[IBIS VER]   4.1
[File Name]   f29h85xrfs.ibs
[File Rev]   1.0
[Date]   May 06, 2024
[Source]   File originated at Texas Instruments
[Copyright]   (c) 2012, Texas Instruments Inc.
[Component]   f29h85xrfs
[Manufacturer]  Texas Instruments
[Package]
| Variable   Typ   Min   Max
R_pkg   2.68E-01   1.13E-01   3.72E-01
L_pkg   6.91E-09   5.05E-09   8.22E-09
C_pkg   1.08E-13   7.65E-14   2.06E-13
[Pin]   signal_name   model_name   R_pin   L_pin   C_pin
1   GPIO15   BQ33100HYPBFZ_PMB_5FS_LC_7LM   2.88E-01   7.82E-09   2.03E-13
2   GPIO16   BCF33100DSHYPBFZ_USF_7LM   2.89E-01   7.74E-09   1.00E-13
3   VDDIO   NC   2.81E-01   7.58E-09   9.82E-14
4   GPIO17   BCF33100DSHYPBFZ_USF_7LM   2.78E-01   7.47E-09   9.65E-14
5   GPIO19   BCF33100DSHYPBFZ_USF_7LM   2.72E-01   7.32E-09   9.48E-14
6   VDD   NC   1.62E-01   6.27E-09   9.54E-14
7   GPIO34   BCF33100DSHYPBFZ_USF_7LM   3.01E-01   7.40E-09   9.18E-14
8   VDD   NC   1.84E-01   6.29E-09   9.29E-14
9   VDDIO   NC   3.72E-01   7.84E-09   8.90E-14
10   GPIO18   BQ33100HYPBFZ_PMB_5FS_LC_7LM   3.58E-01   7.63E-09   8.73E-14
11   GPIO22   BQ33100HYPBFZ_PMB_5FS_LC_7LM   3.52E-01   7.49E-09   8.55E-14
12   B11,GPIO235   BCF33100DSHYPBFZ_USF_7LM   3.46E-01   7.35E-09   8.38E-14
13   B10,GPIO234   BCF33100DSHYPBFZ_USF_7LM   3.33E-01   7.15E-09   8.20E-14
14   B9,GPIO233   BCF33100DSHYPBFZ_USF_7LM   3.33E-01   7.06E-09   8.04E-14
15   B8,GPIO232   BCF33100DSHYPBFZ_USF_7LM   3.22E-01   6.87E-09   7.86E-14
16   A8,GPIO226   BCF33100DSHYPBFZ_USF_7LM   3.17E-01   6.74E-09   7.69E-14
17   A7/E25,GPIO225   BCF33100DSHYPBFZ_USF_7LM   3.23E-01   6.70E-09   2.02E-13
18   A6/E24,GPIO224   BCF33100DSHYPBFZ_USF_7LM   3.12E-01   6.52E-09   1.97E-13
19   VDDA   NC   1.91E-01   5.46E-09   2.00E-13
20   VSSA   NC   1.86E-01   5.50E-09   2.05E-13
21   B5/D31   ICF33SHYPB_LC_7LM   3.28E-01   6.83E-09   7.70E-14
22   B4/D30   ICF33SHYPB_LC_7LM   3.14E-01   6.81E-09   7.85E-14
23   A5/D29   ICF33SHYPB_LC_7LM   3.02E-01   6.78E-09   8.01E-14
24   A4/D28   ICF33SHYPB_LC_7LM   2.90E-01   6.77E-09   8.17E-14
25   B3/D27   ICF33SHYPB_LC_7LM   2.80E-01   6.77E-09   8.32E-14
26   B2/D26   ICF33SHYPB_LC_7LM   2.71E-01   6.79E-09   8.48E-14
27   A3/D25   ICF33SHYPB_LC_7LM   2.64E-01   6.82E-09   8.64E-14
28   A2/D24   ICF33SHYPB_LC_7LM   2.60E-01   6.87E-09   8.81E-14
29   VREFLOAB   NC   1.49E-01   5.99E-09   9.17E-14
30   VREFHIAB   NC   1.13E-01   5.76E-09   9.54E-14
31   A15/B15/C15/D15/E15   ICF33SHYPB_LC_7LM   2.57E-01   7.11E-09   9.30E-14
32   A14/B14/C14/D14/E14   ICF33SHYPB_LC_7LM   2.60E-01   7.22E-09   9.47E-14
33   B1/C27   ICF33SHYPB_LC_7LM   2.65E-01   7.35E-09   9.64E-14
34   B0/C26/VDAC   ICF33SHYPB_LC_7LM   2.72E-01   7.50E-09   9.82E-14
35   A1/C25   ICF33SHYPB_LC_7LM   2.80E-01   7.67E-09   9.99E-14
36   A0/C24/DACA_OUT   ICF33SHYPB_LC_7LM   2.91E-01   7.85E-09   2.03E-13
37   C0/E28   ICF33SHYPB_LC_7LM   2.91E-01   7.89E-09   2.05E-13
38   C1/E29   ICF33SHYPB_LC_7LM   2.80E-01   7.70E-09   1.01E-13
39   D0/B24   ICF33SHYPB_LC_7LM   2.70E-01   7.53E-09   9.89E-14
40   D1/B25   ICF33SHYPB_LC_7LM   2.63E-01   7.38E-09   9.72E-14
41   E0/A24/DACC_OUT   ICF33SHYPB_LC_7LM   2.58E-01   7.24E-09   9.54E-14
42   E1/A25   ICF33SHYPB_LC_7LM   2.55E-01   7.13E-09   9.37E-14
43   C2/E30   ICF33SHYPB_LC_7LM   2.54E-01   7.03E-09   9.20E-14
44   C3/E31   ICF33SHYPB_LC_7LM   2.56E-01   6.96E-09   9.04E-14
45   VREFLOCDE   NC   1.50E-01   5.94E-09   9.08E-14
46   VREFHICDE   NC   1.13E-01   5.52E-09   9.12E-14
47   C4   ICF33SHYPB_LC_7LM   2.67E-01   6.79E-09   8.54E-14
48   C5   ICF33SHYPB_LC_7LM   2.76E-01   6.77E-09   8.38E-14
49   D2/B26   ICF33SHYPB_LC_7LM   2.86E-01   6.77E-09   8.23E-14
50   D3/B27   ICF33SHYPB_LC_7LM   2.97E-01   6.78E-09   8.07E-14
51   E2/A26   ICF33SHYPB_LC_7LM   3.10E-01   6.80E-09   7.91E-14
52   E3/A27   ICF33SHYPB_LC_7LM   3.24E-01   6.83E-09   7.75E-14
53   VSSA   NC   1.84E-01   5.52E-09   2.06E-13
54   VDDA   NC   1.89E-01   5.47E-09   2.02E-13
55   D5/B29,GPIO241   BCF33100DSHYPBFZ_USF_7LM   2.67E-01   6.15E-09   1.98E-13
56   E4/A28,GPIO246   BCF33100DSHYPBFZ_USF_7LM   2.67E-01   6.24E-09   2.03E-13
57   E5/A29,GPIO247   BCF33100DSHYPBFZ_USF_7LM   2.68E-01   6.35E-09   7.71E-14
58   C8,GPIO238   BCF33100DSHYPBFZ_USF_7LM   2.72E-01   6.47E-09   7.88E-14
59   C9,GPIO239   BCF33100DSHYPBFZ_USF_7LM   2.77E-01   6.60E-09   8.05E-14
60   D6/B30,GPIO242   BCF33100DSHYPBFZ_USF_7LM   2.83E-01   6.75E-09   8.22E-14
61   D7/B31,GPIO243   BCF33100DSHYPBFZ_USF_7LM   2.91E-01   6.91E-09   8.40E-14
62   E6/A30,GPIO248   BCF33100DSHYPBFZ_USF_7LM   3.01E-01   7.08E-09   8.57E-14
63   E7/A31,GPIO249   BCF33100DSHYPBFZ_USF_7LM   3.11E-01   7.26E-09   8.75E-14
64   GPIO222/TDI   BCF33100DSHYPBFZ_USF_7LM   3.11E-01   7.35E-09   8.92E-14
65   GPIO223/TDO   BCPF335585DSHYPBFZ_USF_7LM   3.23E-01   7.55E-09   9.10E-14
66   VDDIO   NC   3.35E-01   7.74E-09   9.28E-14
67   VDD   NC   1.42E-01   6.14E-09   1.00E-13
68   VDD3VFL   NC   1.39E-01   6.20E-09   1.01E-13
69   TMS   BCF3355DSHYPBFZ_TMS_USF_7LM   3.36E-01   8.02E-09   9.78E-14
70   TCK   IQ0442FS_40P60P_3X2_USF_7LM   3.49E-01   8.22E-09   9.96E-14
71   VDD   NC   1.47E-01   6.54E-09   1.07E-13
72   VDDIO   NC   2.87E-01   7.86E-09   2.05E-13
73   GPIO41   BCF33100DSHYPBFZ_CORNER_USF_7LM   2.88E-01   7.82E-09   2.03E-13
74   GPIO219/ERRORSTS   BCF33100DSHYPBFZ_CORNER_USF_7LM   3.00E-01   7.84E-09   1.00E-13
75   GPIO49   BCF33100DSHYPBFZ_USF_7LM   2.91E-01   7.67E-09   9.83E-14
76   GPIO50   BCF33100DSHYPBFZ_USF_7LM   2.83E-01   7.52E-09   9.66E-14
77   GPIO51   BCF33100DSHYPBFZ_USF_7LM   2.76E-01   7.37E-09   9.49E-14
78   GPIO52   BCF33100DSHYPBFZ_USF_7LM   2.74E-01   7.26E-09   9.32E-14
79   GPIO53   BCF33100DSHYPBFZ_USF_7LM   2.69E-01   7.12E-09   9.15E-14
80   GPIO54   BCF33100DSHYPBFZ_USF_7LM   2.66E-01   7.01E-09   8.98E-14
81   VDDIO   NC   2.64E-01   6.90E-09   8.81E-14
82   GPIO56   BCF33100DSHYPBFZ_USF_7LM   2.65E-01   6.82E-09   8.64E-14
83   VDD3VFL   NC   1.14E-01   5.41E-09   8.90E-14
84   GPIO57   BCF33100DSHYPBFZ_USF_7LM   2.65E-01   6.65E-09   8.31E-14
85   GPIO58   BCF33100DSHYPBFZ_USF_7LM   2.66E-01   6.56E-09   8.15E-14
86   GPIO59   BCF3385DSHYPBFZ_USF_7LM   2.68E-01   6.49E-09   7.98E-14
87   VDD   NC   1.14E-01   5.05E-09   8.26E-14
88   GPIO60   BCF33100DSHYPBFZ_USF_7LM   2.72E-01   6.35E-09   7.65E-14
89   GPIO61   BCF33100DSHYPBFZ_USF_7LM   2.69E-01   6.23E-09   2.01E-13
90   GPIO62   BCF33100DSHYPBFZ_USF_7LM   2.71E-01   6.16E-09   1.97E-13
91   GPIO63   BCF33100DSHYPBFZ_USF_7LM   2.73E-01   6.18E-09   1.97E-13
92   GPIO64   BCF3385DSHYPBFZ_USF_7LM   2.77E-01   6.30E-09   2.01E-13
93   GPIO65   BCF33100DSHYPBFZ_USF_7LM   2.82E-01   6.43E-09   7.66E-14
94   GPIO66   BCF33100DSHYPBFZ_USF_7LM   2.84E-01   6.54E-09   7.83E-14
95   VDDIO   NC   2.82E-01   6.62E-09   7.99E-14
96   GPIO32   BCF33100DSHYPBFZ_USF_7LM   2.81E-01   6.69E-09   8.16E-14
97   GPIO127   BCF33100DSHYPBFZ_USF_7LM   2.83E-01   6.80E-09   8.33E-14
98   VDD   NC   1.18E-01   5.45E-09   8.93E-14
99   VDDOSC   NC   2.81E-01   6.96E-09   8.66E-14
100   GPIO221,X2   BCPF335585DSHYPBFZ_USF_7LM   2.82E-01   7.06E-09   8.83E-14
101   VSSOSC   NC   2.78E-01   7.12E-09   8.99E-14
102   GPIO220,X1   BCPF335585DSHYPBFZ_USF_7LM   2.88E-01   7.29E-09   9.16E-14
103   XRSn   BQ0491FS_3X2_USF_7LM   2.78E-01   7.29E-09   9.32E-14
104   GPIO38   BCF33100DSHYPBFZ_USF_7LM   2.85E-01   7.44E-09   9.49E-14
105   GPIO103   BCF33100DSHYPBFZ_USF_7LM   2.93E-01   7.60E-09   9.67E-14
106   VDDIO   NC   2.96E-01   7.72E-09   9.84E-14
107   GPIO42   BCPF335585DSHYPBFZ_USF_7LM   2.89E-01   7.74E-09   1.00E-13
108   GPIO43   BCF33100DSHYPBFZ_CORNER_USF_7LM   2.98E-01   7.91E-09   2.03E-13
109   GPIO68   BCF33100DSHYPBFZ_CORNER_USF_7LM   2.87E-01   7.86E-09   2.05E-13
110   GPIO70   BCF3385DSHYPBFZ_CORNER_7LM   2.88E-01   7.77E-09   1.01E-13
111   GPIO71   BCF33100DSHYPBFZ_USF_7LM   2.79E-01   7.61E-09   9.90E-14
112   VDD   NC   1.61E-01   6.48E-09   9.94E-14
113   VDDIO   NC  2.85E-01  7.48E-09  9.57E-14
114   GPIO72   BCF33100DSHYPBFZ_USF_7LM   2.77E-01   7.32E-09   9.39E-14
115   GPIO76   BCF33100DSHYPBFZ_USF_7LM   2.86E-01   7.31E-09   9.23E-14
116   GPIO77   BCF33100DSHYPBFZ_USF_7LM   2.78E-01   7.15E-09   9.06E-14
117   GPIO78   BCF33100DSHYPBFZ_USF_7LM   2.72E-01   7.00E-09   8.88E-14
118   VDDIO   NC   2.70E-01   6.90E-09   8.71E-14
119   GPIO84   BCF33100DSHYPBFZ_USF_7LM   2.76E-01   6.86E-09   8.55E-14
120   GPIO30   BCF3355DSHYPBFZ_USF_7LM   2.93E-01   6.92E-09   8.40E-14
121   GPIO29   BQ33100HYPBFZ_PMB_5FS_LC_7LM   2.93E-01   6.83E-09   8.23E-14
122   VDDIO   NC   2.90E-01   6.71E-09   8.06E-14
123   VDD   NC   1.60E-01   5.49E-09   8.12E-14
124   GPIO26   BCF33100DSHYPBFZ_USF_7LM   2.96E-01   6.59E-09   7.73E-14
125   GPIO25   BCF33100DSHYPBFZ_USF_7LM   2.88E-01   6.43E-09   2.03E-13
126   GPIO24   BCF33100DSHYPBFZ_USF_7LM   2.81E-01   6.28E-09   1.98E-13
127   GPIO23   BQ33100HYPBFZ_PMB_5FS_LC_7LM   2.76E-01   6.24E-09   1.98E-13
128   GPIO0   BCF33100DSHYPBFZ_USF_7LM   2.79E-01   6.35E-09   2.03E-13
129   GPIO1   BCF33100DSHYPBFZ_USF_7LM   2.73E-01   6.38E-09   7.71E-14
130   GPIO2   BCF33100DSHYPBFZ_USF_7LM   2.68E-01   6.43E-09   7.87E-14
131   GPIO3   BCF33100DSHYPBFZ_USF_7LM   2.65E-01   6.49E-09   8.04E-14
132   GPIO4   BCF33100DSHYPBFZ_USF_7LM   2.63E-01   6.57E-09   8.21E-14
133   GPIO5   BCF33100DSHYPBFZ_USF_7LM   2.63E-01   6.66E-09   8.37E-14
134   GPIO6   BCF3355DSHYPBFZ_USF_7LM   2.64E-01   6.76E-09   8.54E-14
135   GPIO7   BCF33100DSHYPBFZ_USF_7LM   2.65E-01   6.85E-09   8.71E-14
136   VDDIO   NC   2.66E-01   6.96E-09   8.88E-14
137   VDD   NC   1.62E-01   6.14E-09   9.29E-14
138   GPIO8   BCF33100DSHYPBFZ_USF_7LM   2.68E-01   7.15E-09   9.22E-14
139   GPIO9   BCF3385DSHYPBFZ_USF_7LM   2.74E-01   7.30E-09   9.39E-14
140   GPIO10   BQ33100HYPBFZ_PMB_5FS_LC_7LM   2.73E-01   7.38E-09   9.56E-14
141   GPIO11   BCF33100DSHYPBFZ_USF_7LM   2.76E-01   7.49E-09   9.73E-14
142   GPIO12   BCF33100DSHYPBFZ_CORNER_USF_7LM   2.79E-01   7.61E-09   9.90E-14
143   GPIO13   BCF33100DSHYPBFZ_USF_7LM   2.83E-01   7.73E-09   1.01E-13
144   GPIO14   BCF33100DSHYPBFZ_CORNER_USF_7LM   2.89E-01   7.87E-09   2.05E-13
| End of package information
|   Component BCF33100DSHYPBFZ_7LM
[Component]   BCF33100DSHYPBFZ_7LM
[Manufacturer]  IO Methodology Inc.
[Package]
|   typ   min   max
R_pkg   0   0   0
L_pkg   0   0   0
C_pkg   0   0   0
[Pin]   signal_name  model_name   R_pin   L_pin   C_pin
VSS   VSS   GND
VDDS   VDDS   POWER
PAD   PAD   BCF33100DSHYPBFZ_7LM
[Model Selector] BCF33100DSHYPBFZ_7LM
WK_PU_ON_3P3  Cell operated at 3.3(nom)
|WK_PU_ON_3P3; WEAK_PULLUP_ON
WK_PD_ON_3P3  Cell operated at 3.3(nom)
|WK_PD_ON_3P3; WEAK_PULLDOWN_ON
DRIVER_MODE_3P3  Cell operated at 3.3(nom)
|DRIVER_MODE_3P3
RECEIVER_MODE_3P3  Cell operated at 3.3(nom)
|   Component BCF33100DSHYPBFZ_USF_7LM
[Component]   BCF33100DSHYPBFZ_USF_7LM
[Manufacturer]  Texas Instruments
[Package]
| variable   typ   min   max
R_pkg   0.0   0.0   0.0
L_pkg   0.0H   0.0H   0.0H
C_pkg   0.0F   0.0F   0.0F
[Pin]  signal_name   model_name   R_pin   L_pin   C_pin
PAD   PAD   BCF33100_USF_7LM_IO_3.3V   0   0   0
VDDS   VDDS   Power   0   0   0
VSS   VSS   Gnd   0   0   0
[Model Selector] BCF33100DSHYPBFZ_USF_7LM
BCF33100_USF_7LM_IO_3.3V I/O model with 3.3V supply
|   Component BCF33100DSHYPBFZ_CORNER_USF_7LM
[Component]   BCF33100DSHYPBFZ_CORNER_USF_7LM
[Manufacturer]  Texas Instruments
[Package]
| variable   typ   min   max
R_pkg   0.0   0.0   0.0
L_pkg   0.0H   0.0H   0.0H
C_pkg   0.0F   0.0F   0.0F
[Pin]  signal_name   model_name   R_pin   L_pin   C_pin
PAD   PAD   BCF33100_CORNER_7LM_IO_3.3V   0   0   0
VDDS   VDDS   Power   0   0   0
VSS   VSS   Gnd   0   0   0
[Model Selector] BCF33100DSHYPBFZ_CORNER_USF_7LM
BCF33100_CORNER_7LM_IO_3.3V  I/O model with 3.3V supply
|   Component BCF3355DSHYPBFZ_TMS_USF_7LM
[Component]   BCF3355DSHYPBFZ_TMS_USF_7LM
[Manufacturer]  Texas Instruments
[Package]
| variable   typ   min   max
R_pkg   0.0   0.0   0.0
L_pkg   0.0H   0.0H   0.0H
C_pkg   0.0F   0.0F   0.0F
[Pin]  signal_name   model_name   R_pin   L_pin   C_pin
PAD   PAD   BCF3355_TMS_7LM_IO_3.3V   0   0   0
VDDS   VDDS   Power   0   0   0
VSS   VSS   Gnd   0   0   0
[Model Selector] BCF3355DSHYPBFZ_TMS_USF_7LM
BCF3355_TMS_7LM_IO_3.3V I/O model with 3.3V supply
|   Component IQ0442FS_40P60P_3X2_USF_7LM
[Component]   IQ0442FS_40P60P_3X2_USF_7LM
[Manufacturer]  Texas Instruments
[Package]
| variable   typ   min   max
R_pkg   0.0   0.0   0.0
L_pkg   0.0H   0.0H   0.0H
C_pkg   0.0F   0.0F   0.0F
[Pin]  signal_name   model_name   R_pin   L_pin   C_pin
PAD   PAD   IQRX_3.3V   0   0   0
VDDS   VDDS   Power   0   0   0
VSS   VSS   Gnd   0   0   0
[Model Selector] IQ0442FS_40P60P_3X2_USF_7LM
IQRX_3.3V I/O model with 3.3V supply
|   Component BCF3355DSHYPBFZ_USF_7LM
[Component]   BCF3355DSHYPBFZ_USF_7LM
[Manufacturer]  Texas Instruments
[Package]
| variable   typ   min   max
R_pkg   0.0   0.0   0.0
L_pkg   0.0H   0.0H   0.0H
C_pkg   0.0F   0.0F   0.0F
[Pin]  signal_name   model_name   R_pin   L_pin   C_pin
PAD   PAD   BCF3355_USF_7LM_IO_3.3V   0   0   0
VDDS   VDDS   Power   0   0   0
VSS   VSS   Gnd   0   0   0
[Model Selector] BCF3355DSHYPBFZ_USF_7LM
BCF3355_USF_7LM_IO_3.3V I/O model with 3.3V supply
|   Component BCF3385DSHYPBFZ_CORNER_7LM
[Component]   BCF3385DSHYPBFZ_CORNER_7LM
[Manufacturer]  IO Methodology Inc.
[Package]
|   typ   min   max
R_pkg   0   0   0
L_pkg   0   0   0
C_pkg   0   0   0
[Pin]   signal_name  model_name   R_pin   L_pin   C_pin
VSS   VSS   GND
VDDS   VDDS   POWER
PAD   PAD   BCF3385DSHYPBFZ_CORNER_7LM
[Model Selector] BCF3385DSHYPBFZ_CORNER_7LM
WK_PU_ON_3P3_BCF3385DSHYPBFZ_CORNER_7LM  Cell operated at 3.3(nom)
|WK_PU_ON_3P3; WEAK_PULLUP_ON
WK_PD_ON_3P3_BCF3385DSHYPBFZ_CORNER_7LM  Cell operated at 3.3(nom)
|WK_PD_ON_3P3; WEAK_PULLDOWN_ON
DRIVER_MODE_3P3_BCF3385_CORNER_7LM Cell operated at 3.3(nom)
|DRIVER_MODE_3P3
RECEIVER_MODE_3P3_BCF3385_CORNER_7LM  Cell operated at 3.3(nom)
|   Component BCF3385DSHYPBFZ_USF_7LM
[Component]   BCF3385DSHYPBFZ_USF_7LM
[Manufacturer]  Texas Instruments
[Package]
| variable   typ   min   max
R_pkg   0.0   0.0   0.0
L_pkg   0.0H   0.0H   0.0H
C_pkg   0.0F   0.0F   0.0F
[Pin]  signal_name   model_name   R_pin   L_pin   C_pin
PAD   PAD   BCF3385_USF_7LM_IO_3.3V   0   0   0
VDDS   VDDS   Power   0   0   0
VSS   VSS   Gnd   0   0   0
[Model Selector] BCF3385DSHYPBFZ_USF_7LM
BCF3385_USF_7LM_IO_3.3V I/O model with 3.3V supply
|   Component BCPF335585DSHYPBFZ_USF_7LM
[Component]   BCPF335585DSHYPBFZ_USF_7LM
[Manufacturer]  Texas Instruments
[Package]
| variable   typ   min   max
R_pkg   0.0   0.0   0.0
L_pkg   0.0H   0.0H   0.0H
C_pkg   0.0F   0.0F   0.0F
[Pin]  signal_name   model_name   R_pin   L_pin   C_pin
PAD   PAD   BCPF335585DSHYPBFZ_USF_7LM   0   0   0
VDDS   VDDS   Power   0   0   0
VSS   VSS   Gnd   0   0   0
[Model Selector]   BCPF335585DSHYPBFZ_USF_7LM
BCPF335585_7LM_IO_DS0_3.3V   I/O model DS 0 with 3.3V supply
BCPF335585_7LM_IO_DS1_3.3V   I/O model DS 1 with 3.3V supply
|   Component BQ0491FS_3X2_USF_7LM
[Component]   BQ0491FS_3X2_USF_7LM
[Manufacturer]  Texas Instruments
[Package]
| variable   typ   min   max
R_pkg   0.0   0.0   0.0
L_pkg   0.0H   0.0H   0.0H
C_pkg   0.0F   0.0F   0.0F
[Pin]  signal_name   model_name   R_pin   L_pin   C_pin
PAD   PAD   BQ0491FS_3X2_USF_7LM   0   0   0
VDDS   VDDS   Power   0   0   0
VSS   VSS   Gnd   0   0   0
[Model Selector]   BQ0491FS_3X2_USF_7LM
BQ0491_3X2_USF_7LM_IO_15p_3p3   I/O open drain model with C_fixture 15pF for 3.3V supply
BQ0491_3X2_USF_7LM_IO_50p_3p3   I/O open drain model with C_fixture 50pF for 3.3V supply
BQ0491_3X2_USF_7LM_IO_100p_3p3   I/O open drain model with C_fixture 100pF for 3.3V supply
BQ0491_3X2_USF_7LM_IO_150p_3p3   I/O open drain model with C_fixture 150pF for 3.3V supply
|   Component BQ33100HYPBFZ_PMB_5FS_LC_7LM
[Component]   BQ33100HYPBFZ_PMB_5FS_LC
[Manufacturer]  Texas Instruments
[Package]
| variable   typ   min   max
R_pkg   0.0   0.0   0.0
L_pkg   0.0H   0.0H   0.0H
C_pkg   0.0F   0.0F   0.0F
[Pin]  signal_name   model_name   R_pin   L_pin   C_pin
Pin1   PAD   BQ33100HYPBFZ_PMB_5FS_LC_7LM   0   0   0
Pin2   VDDS   Power   0   0   0
Pin3   VSS   Gnd   0   0   0
[Model Selector]   BQ33100HYPBFZ_PMB_5FS_LC_7LM
BQ33_PMB_IO_M0_D0   I/O model with Mode = 0 and Drive = 0
BQ33_PMB_IO_M0_D1   I/O model with Mode = 0 and Drive = 1
BQ33_PMB_IO_M1_D0   I/O model with Mode = 1 and Drive = 0
BQ33_PMB_IO_M1_D1   I/O model with Mode = 1 and Drive = 1
|   Component IQ0440FS_VREGENZ_PU_7LM
[Component]   IQ0440FS_VREGENZ_PU_7LM
[Manufacturer]  Texas Instruments
[Package]
|   typ   min   max
R_pkg   0   0   0
L_pkg   0   0   0
C_pkg   0   0   0
[Pin]   signal_name  model_name   R_pin   L_pin   C_pin
VSS   VSS   GND
VDDS   VDDS   POWER
PAD   PAD   IQ0440FS_VREGENZ_PU_7LM
[Model Selector] IQ0440FS_VREGENZ_PU_7LM
WK_PD_ON_3P3_IQ0440FS_VREGENZ_PU_7LM Cell operated at 3.3(nom)
|WK_PD_ON_3P3; WEAK_PULLDOWN_ON
RECEIVER_MODE_3P3_IQ0440FS_VREGENZ  Cell operated at 3.3(nom)
|   Component ICF33SHYPB_LC_7LM
[Component]   ICF33SHYPB_LC_7LM
[Manufacturer]   Texas Instruments
[Package]
|  variable   typ   min   max
R_pkg   0   0   0
L_pkg   0   0   0
C_pkg   0   0   0
[Pin]   signal_name   model_name   R_pin   L_pin   C_pin
VSS   VSS   GND
VDDS   VDDS   POWER
PAD   PAD   ICF33SHYPB_LC_7LM
[Model Selector] ICF33SHYPB_LC_7LM
RECEIVER_MODE_3P3_ICF_7LM  Cell operated at 3.3(nom)
|RECEIVER_MODE_3P3_ICF_7LM; RECEIVER_MODE
WK_PU_ON_3P3_ICF_7LM  Cell operated at 3.3(nom)
|WK_PU_ON_3P3_ICF_7LM; WEAK_PULLUP_ON
WK_PD_ON_3P3_ICF_7LM  Cell operated at 3.3(nom)
| Models and submodels in the file (29): WK_PU_ON_3P3 (Input), WK_PD_ON_3P3 (Input), DRIVER_MODE_3P3 (I/O), RECEIVER_MODE_3P3 (Input), BCF33100_USF_7LM_IO_3.3V (I/O), BCF33100_CORNER_7LM_IO_3.3V (I/O), BCF3355_TMS_7LM_IO_3.3V (I/O), IQRX_3.3V (Input), BCF3355_USF_7LM_IO_3.3V (I/O), WK_PU_ON_3P3_BCF3385DSHYPBFZ_CORNER_7LM (Input), WK_PD_ON_3P3_BCF3385DSHYPBFZ_CORNER_7LM (Input), DRIVER_MODE_3P3_BCF3385_CORNER_7LM (I/O), RECEIVER_MODE_3P3_BCF3385_CORNER_7LM (Input), BCF3385_USF_7LM_IO_3.3V (I/O), BCPF335585_7LM_IO_DS0_3.3V (I/O), BCPF335585_7LM_IO_DS1_3.3V (I/O), BQ0491_3X2_USF_7LM_IO_15p_3p3 (I/O_open_drain), BQ0491_3X2_USF_7LM_IO_50p_3p3 (I/O_open_drain), BQ0491_3X2_USF_7LM_IO_100p_3p3 (I/O_open_drain), BQ0491_3X2_USF_7LM_IO_150p_3p3 (I/O_open_drain), BQ33_PMB_IO_M0_D0 (I/O), BQ33_PMB_IO_M0_D1 (I/O), BQ33_PMB_IO_M1_D0 (I/O), BQ33_PMB_IO_M1_D1 (I/O), WK_PD_ON_3P3_IQ0440FS_VREGENZ_PU_7LM (Input), RECEIVER_MODE_3P3_IQ0440FS_VREGENZ (Input), RECEIVER_MODE_3P3_ICF_7LM (Input), WK_PU_ON_3P3_ICF_7LM (Input), WK_PD_ON_3P3_ICF_7LM (Input)
